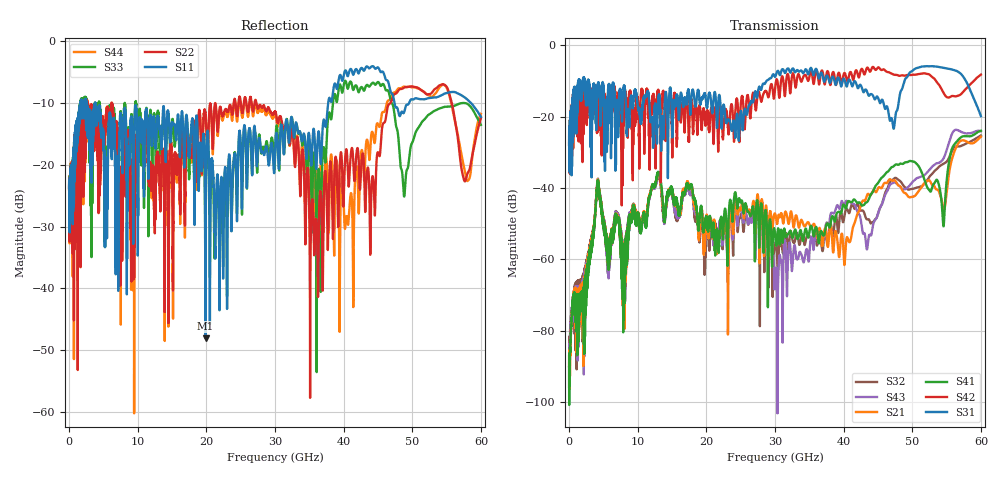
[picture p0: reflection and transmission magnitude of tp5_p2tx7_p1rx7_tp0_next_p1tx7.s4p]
! 100G CR Analysis
! File: tp5_p2tx7_p1rx7_tp0_next_p1tx7
! Description: 2m Cu Cable, OSFP, TP0-TP5
! Port Mapping
! Port1 -- P1RX7N
! Port2 -- P1TX7N
! Port3 -- P1RX7P
! Port4 -- P1TX7P
# GHz S MA R 50.00
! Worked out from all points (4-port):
!   6000 points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, 10 MHz to 60 GHz, reference 50 ohm
!   strongest paths, dB at 10 MHz, 15.01 GHz, 30.01 GHz, 45.01 GHz, 60 GHz:
!     S31: -27.9, -21.7, -8.9, -14.7, -19.9
!     S42: -27.9, -26.0, -12.2, -6.2, -8.2
!     S41: -90.2, -41.1, -52.7, -38.6, -24.0
!     S21: -87.2, -41.4, -47.2, -40.1, -25.6
!     S43: -95.8, -41.8, -66.9, -47.1, -24.1
!     S32: -89.9, -42.2, -56.1, -47.4, -25.3
!   lowest |S11| = -48.0 dB at 19.88 GHz (marker M1), VSWR 1.01, Z = 50 - j0.394 ohm
!   |S11| at or under -10 dB: start of sweep to 1.64 GHz; 3.811 GHz to 37.76 GHz (33.95 GHz wide, 163 % of centre); 47.4 GHz to 49.56 GHz (2.156 GHz wide, 4.45 % of centre)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
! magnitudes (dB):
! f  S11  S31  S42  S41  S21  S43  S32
! 10 MHz  -23.7  -27.9  -27.9  -90.2  -87.2  -95.8  -89.9
! 4.22 GHz  -11.2  -10.6  -12.3  -38.3  -38.2  -38.1  -38.0
! 7.94 GHz  -14.0  -11.9  -18.2  -77.0  -75.1  -74.4  -71.0
! 19.88 GHz  -48.0  -14.4  -22.6  -49.0  -51.1  -53.7  -56.8
! 30.19 GHz  -14.9  -8.0  -9.8  -56.2  -48.8  -62.6  -55.3
! 36.03 GHz  -20.6  -6.6  -6.9  -51.0  -53.0  -52.5  -55.4
! 60 GHz  -12.3  -19.9  -8.2  -24.0  -25.6  -24.1  -25.3
